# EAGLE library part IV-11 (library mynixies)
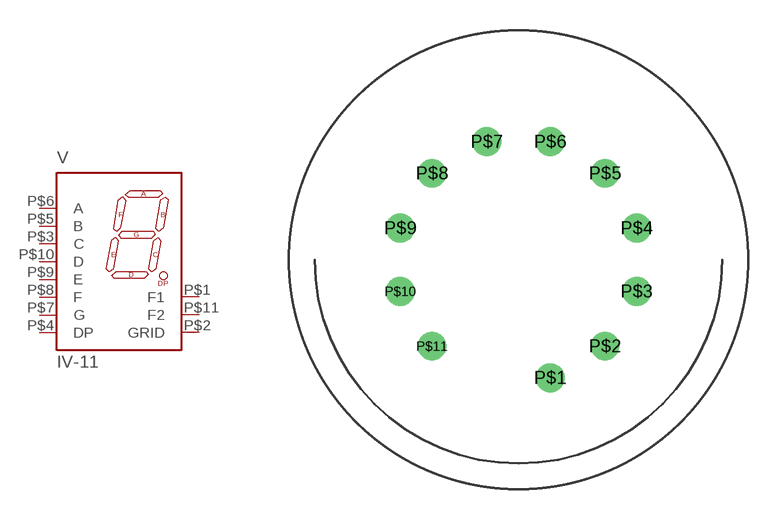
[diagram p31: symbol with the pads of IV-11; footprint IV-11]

Designator prefix V

## IV-11  [IV-11]
P$1  F1  pas
P$2  GRID  pas
P$3  C  pas
P$4  DP  pas
P$5  B  pas
P$6  A  pas
P$7  G  pas
P$8  F  pas
P$9  E  pas
P$10  D  pas
P$11  F2  pas

## Footprint IV-11 (pad centres in mm)
drill 0.9: P$1 1.553,-5.796; P$2 4.243,-4.243; P$3 5.796,-1.553; P$4 5.796,1.553; P$5 4.243,4.243; P$6 1.553,5.796; P$7 -1.553,5.796; P$8 -4.243,4.243; P$9 -5.796,1.553; P$10 -5.796,-1.553; P$11 -4.243,-4.243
